// ------------------------------------------------------------------
// File           : D:\WZVBSP\WZV_VAR.AWL
//
// Source File    : D:\WZVBSP\WZV_VAR.VAR
// Generation Date: 05-August-99  Time: 08:38
// ------------------------------------------------------------------

DATA_BLOCK DB  119
VERSION : 0.0


STRUCT

 N_Y_numMagPlaceParams_27:
   STRUCT
   SYNTAX_ID : BYTE  := B#16#82;
   bereich_u_einheit :byte := B#16#1;
   spalte :word := W#16#1B;
   zeile :word := W#16#1;
   bausteintyp :byte := B#16#10;
   ZEILENANZAHL : BYTE := B#16#1;
   typ :byte := B#16#4;
   laenge :byte := B#16#2;
   END_STRUCT ;

 T0_TP_placeData0_0:
   STRUCT
   SYNTAX_ID : BYTE  := B#16#82;
   bereich_u_einheit :byte := B#16#80;
   spalte :word := W#16#0;
   zeile :word := W#16#0;
   bausteintyp :byte := B#16#28;
   ZEILENANZAHL : BYTE := B#16#1;
   typ :byte := B#16#4;
   laenge :byte := B#16#2;
   END_STRUCT ;

 T0_TMC_magCBCmd1_0:
   STRUCT
   SYNTAX_ID : BYTE  := B#16#82;
   bereich_u_einheit :byte := B#16#80;
   spalte :word := W#16#0;
   zeile :word := W#16#1;
   bausteintyp :byte := B#16#2C;
   ZEILENANZAHL : BYTE := B#16#1;
   typ :byte := B#16#4;
   laenge :byte := B#16#2;
   END_STRUCT ;

 T0_TD_toolState0_0:
   STRUCT
   SYNTAX_ID : BYTE  := B#16#82;
   bereich_u_einheit :byte := B#16#80;
   spalte :word := W#16#0;
   zeile :word := W#16#0;
   bausteintyp :byte := B#16#21;
   ZEILENANZAHL : BYTE := B#16#1;
   typ :byte := B#16#4;
   laenge :byte := B#16#2;
   END_STRUCT ;

 END_STRUCT ;

BEGIN
END_DATA_BLOCK
